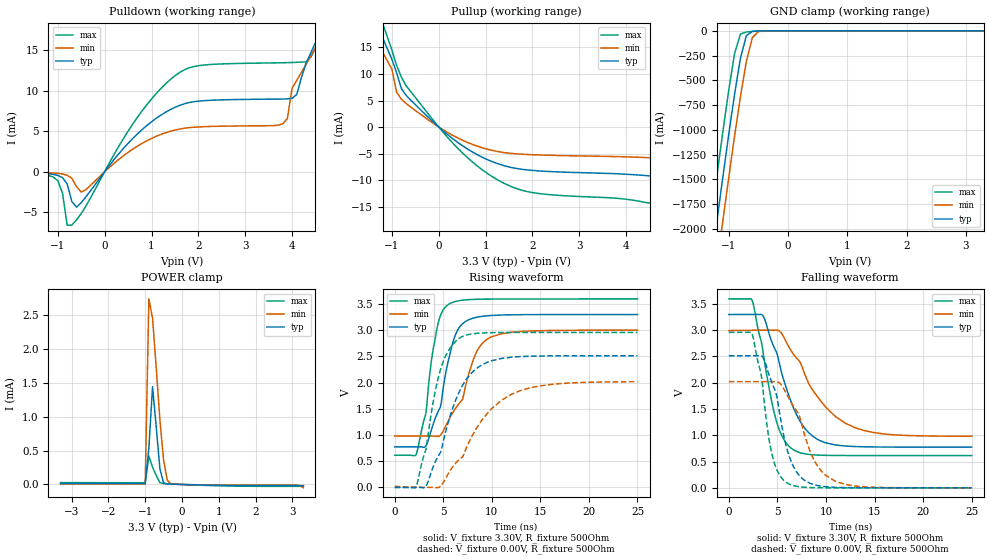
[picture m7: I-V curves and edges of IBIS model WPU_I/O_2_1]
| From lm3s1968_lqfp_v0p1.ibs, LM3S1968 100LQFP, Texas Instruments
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[Model]   WPU_I/O_2_1
Model_type   I/O
Vinl = 1.26
Vinh = 2.04
Vmeas = 1.65
| variable   typ   min   max
C_comp   9.739pF   9.739pF   9.739pF
[Model Spec]
Vinh+   1.91   1.78   2.04
Vinh-   1.90   1.76   2.03
Vinl+   1.40   1.27   1.54
Vinl-   1.39   1.26   1.53
| variable   typ   min   max
[Temperature Range]  25   85   -40
[Voltage Range]   3.3V   3.0V   3.6V
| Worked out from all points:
|   slope of the pulldown table from 0 to 0.495 V, typ, clamps not added: 143 ohm
|   slope of the pullup table from 0 to 0.495 V, typ, clamps not added: 143 ohm
|   GND clamp passes 1 mA (typ) near -0.48 V on its own axis
|   POWER clamp passes 1 mA (typ) near -0.73 V on its own axis
|   falling waveform, V_fixture 3.30V, R_fixture 500Ohm: 20-80 % time 2.91ns typ, 4.35ns min, 1.96ns max; typ from 3.29 V to 0.774 V
|   rising waveform, V_fixture 3.30V, R_fixture 500Ohm: 20-80 % time 1.93ns typ, 2.62ns min, 1.41ns max; typ from 0.774 V to 3.3 V
|   falling waveform, V_fixture 0.00V, R_fixture 500Ohm: 20-80 % time 2ns typ, 2.73ns min, 1.46ns max; typ from 2.51 V to 0 V
|   rising waveform, V_fixture 0.00V, R_fixture 500Ohm: 20-80 % time 2.98ns typ, 4.63ns min, 1.95ns max; typ from 0.002 V to 2.51 V
[Pulldown]
|  Voltage   I(typ)   I(min)   I(max)
-3.3V     -63.97uA   -36.29uA   -90.89uA
-1.1V     -317.2uA   -146.3uA   -639.6uA
-700mV    -3.674mA   -802.3uA   -6.561mA
-500mV    -3.8mA     -2.497mA   -5.141mA
600mV     4.106mA    2.793mA    5.879mA
1.5V      7.937mA    5.14mA     11.83mA
3.8V      8.962mA    5.903mA    13.43mA
4.1V      9.518mA    11.26mA    13.48mA
4.6V      17.2mA     16.24mA    17.2mA
4.8V      19.76mA    18.22mA    20.43mA
6.5V      43.78mA    32.33mA    51.9mA
6.6V      45.47mA    7.61mA     54.43mA
[Pullup]
|  Voltage   I(typ)   I(min)   I(max)
-3.3V     58.76mA    44.69mA    74.9mA
-1.5V     22.87mA    18.92mA    27.05mA
-1.3V     18.86mA    15.72mA    22.09mA
-1.2V     16.83mA    14.11mA    19.57mA
-1V       12.74mA    10.89mA    14.48mA
-900mV    10.18mA    6.552mA    11.57mA
-600mV    5.084mA    3.776mA    6.691mA
500mV     -3.481mA   -2.455mA   -4.825mA
1.5V      -7.517mA   -4.915mA   -11.03mA
5V        -9.793mA   -6.102mA   -15.25mA
5.9V      -11.98mA   -7.296mA   -18.76mA
6.6V      -15.07mA   -8.994mA   -23.96mA
[GND Clamp]
|  Voltage   I(typ)   I(min)   I(max)
-3.3V     -11.72A    -12.12A    -11.3A
-1.4V     -2.845A    -3.285A    -2.387A
-1.3V     -2.39A     -2.831A    -1.93A
-1.2V     -1.938A    -2.38A     -1.478A
-1.1V     -1.494A    -1.934A    -1.036A
-1V       -1.059A    -1.496A    -610.6mA
-900mV    -645mA     -1.069A    -232.9mA
-800mV    -277.1mA   -664.4mA   -31.6mA
-700mV    -48.56mA   -306.6mA   -12.11mA
-600mV    -5.565mA   -70.2mA    -6.295mA
-500mV    -1.181mA   -7.883mA   -2.191mA
3.3V      2.282nA    6.919uA    -6.845uA
[POWER Clamp]
|  Voltage   I(typ)   I(min)   I(max)
-3.3V     15.18uA    8.315uA    27.48uA
-1V       14.14uA    7.74uA     25.63uA
-900mV    539.2uA    2.746mA    419.4uA
-800mV    1.446mA    2.463mA    255uA
-700mV    851uA      1.726mA    135.8uA
-600mV    231.3uA    957.3uA    27.23uA
-500mV    21.69uA    361.2uA    14.14uA
-400mV    7.764uA    63.51uA    10.49uA
-300mV    5.5uA      6.919uA    7.727uA
3.1V      -16.64uA   -9.947uA   -27.43uA
3.2V      -16.65uA   -12.11uA   -27.44uA
3.3V      -16.65uA   -49.87uA   -27.45uA
[Ramp]
| variable   typ   min   max
dV/dt_f   1.51/2.91n   1.20/4.35n   1.79/1.96n
dV/dt_r   1.50/2.98n   1.20/4.63n   1.77/1.95n
R_load = 500Ohm
[Falling Waveform]
V_fixture = 3.30V
V_fixture_min = 3.00V
V_fixture_max = 3.60V
R_fixture = 500Ohm
|   Time   V(typ)   V(min)   V(max)
0s        3.294V     2.989V     3.591V
2.4ns     3.295V     2.995V     3.563V
3.5ns     3.274V     2.996V     2.613V
4.8ns     2.619V     2.997V     1.334V
5.6ns     2.08V      2.885V     940.5mV
6.6ns     1.546V     2.554V     729.4mV
8.9ns     947.9mV    1.79V      624.9mV
11ns      814.5mV    1.352V     615.6mV
13ns      784.5mV    1.143V     614.4mV
25ns      774.3mV    980.8mV    614.1mV
[Rising Waveform]
V_fixture = 3.30V
V_fixture_min = 3.00V
V_fixture_max = 3.60V
R_fixture = 500Ohm
|   Time   V(typ)   V(min)   V(max)
0s        774.3mV    980mV      614.1mV
2.2ns     774.3mV    980mV      626.1mV
3.2ns     789.7mV    979.9mV    1.403V
3.7ns     1.052V     980mV      2.304V
4.4ns     1.419V     972.8mV    3.071V
5.6ns     2.479V     1.3V       3.495V
6.9ns     3.104V     1.656V     3.567V
8.3ns     3.238V     2.531V     3.585V
9.9ns     3.277V     2.865V     3.59V
25ns      3.296V     2.998V     3.594V
[Falling Waveform]
V_fixture = 0.00V
V_fixture_min = 0.00V
V_fixture_max = 0.00V
R_fixture = 500Ohm
|   Time   V(typ)   V(min)   V(max)
0s        2.51V      2.018V     2.956V
2.4ns     2.51V      2.018V     2.925V
3.3ns     2.51V      2.018V     2.184V
4.4ns     2.016V     2.018V     673.6mV
4.9ns     1.771V     2.018V     362.9mV
6ns       729mV      1.764V     94.22mV
7.7ns     157.1mV    1.076V     12.63mV
9.1ns     45.94mV    426.2mV    2.651mV
11ns      9.193mV    121.6mV    418.3uV
25ns      27.86uV    63.93uV    19.33uV
[Rising Waveform]
V_fixture = 0.00V
V_fixture_min = 0.00V
V_fixture_max = 0.00V
R_fixture = 500Ohm
|   Time   V(typ)   V(min)   V(max)
0s        2.209mV    22.16mV    122.4uV
2.2ns     370.3uV    5.824mV    15.24mV
3.2ns     18.81mV    3.22mV     714.1mV
4ns       412mV      1.785mV    1.669V
4.7ns     662mV      19.48mV    2.238V
5.5ns     1.235V     257.7mV    2.598V
6.7ns     1.843V     541.5mV    2.851V
8.7ns     2.303V     1.208V     2.94V
12ns      2.483V     1.774V     2.954V
25ns      2.51V      2.016V     2.955V
